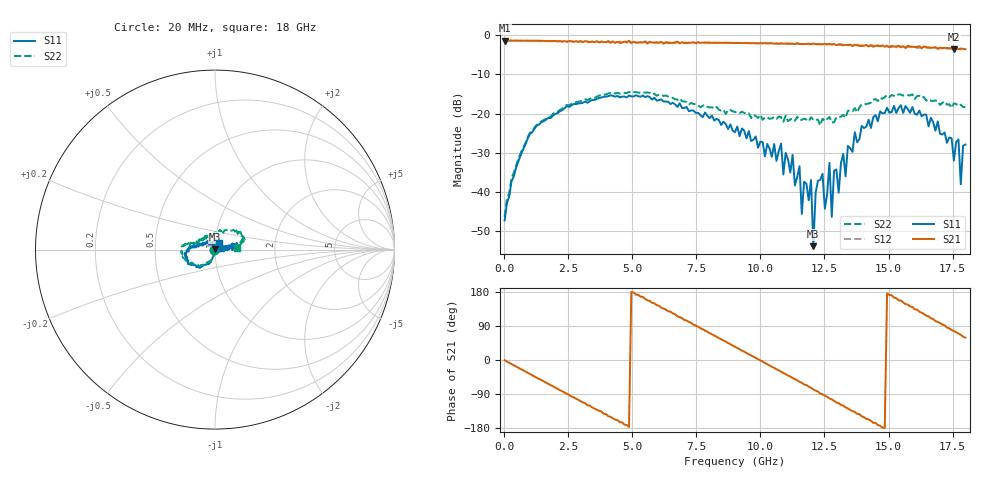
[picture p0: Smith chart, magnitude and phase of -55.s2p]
!Agilent Technologies,N5230A,US43500223,A.07.50.48
!Agilent N5230A: A.07.50.48
!Date: Sunday, January 31, 2016 13:36:31
!Correction: S11(Full 2 Port(1,2))
!S21(Full 2 Port(1,2))
!S12(Full 2 Port(1,2))
!S22(Full 2 Port(1,2))
!S2P File: Measurements: S11, S21, S12, S22:
# Hz S  RI  R 50
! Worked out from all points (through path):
!   201 points, 20 MHz to 18 GHz, reference 50 ohm
!   highest |S21| = -1.32 dB at 20 MHz (marker M1); lowest = -3.6 dB at 17.55 GHz (marker M2)
!   group delay of S21, straight-line fit = 102 ps
!   lowest |S11| = -53.9 dB at 12.07 GHz (marker M3), VSWR 1.00, Z = 49.8 + j0.117 ohm
!   |S11| at or under -10 dB: start of sweep to end of sweep
!   |S22| runs from -46.4 to -14.5 dB; largest |S21 - S12| = 0.077
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2e7  -0.00349 -0.0025  0.859 -0.0113  0.8605 -0.0142  -0.00469 -0.00101
1.0089e9  -0.0166 -0.0525  0.678 -0.5131  0.6764 -0.5149  -0.0171 -0.0541
3.0766e9  -0.0983 -0.0962  -0.3064 -0.759  -0.3201 -0.7628  -0.1247 -0.0772
6.0433e9  -0.1483 0.00658  -0.6466 0.4833  -0.6178 0.4968  -0.1726 0.0232
9.01e9  -0.0414 0.0401  0.6563 0.4582  0.6744 0.4338  -0.0957 0.0436
1.12575e10  0.0141 0.0261  0.5291 -0.5742  0.4974 -0.6035  -0.0459 0.0728
1.15272e10  -0.000936 0.0212  0.4165 -0.6539  0.3888 -0.6794  -0.0414 0.0714
1.16171e10  4.4e-05 0.0052  0.384 -0.6723  0.3423 -0.69  -0.0471 0.0684
1.19767e10  0.013 0.00541  0.2195 -0.739  0.1854 -0.7496  -0.0458 0.0773
1.20666e10  -0.00163 0.00118  0.167 -0.7685  0.1321 -0.7647  -0.0353 0.0753
1.22464e10  0.0124 0.00601  0.0891 -0.7691  0.0505 -0.7681  -0.0333 0.077
1.25161e10  -0.000176 0.00605  -0.0569 -0.7774  -0.0881 -0.7602  -0.0187 0.0779
1.26959e10  0.0201 -0.0121  -0.1503 -0.7608  -0.1919 -0.7475  -0.0232 0.0874
1.27858e10  0.00386 0.00279  -0.1849 -0.7414  -0.2245 -0.7286  -0.0151 0.075
1.28757e10  0.0066 -0.0173  -0.234 -0.7376  -0.2664 -0.7209  -0.0115 0.0769
1.30555e10  0.00962 0.00125  -0.3079 -0.7032  -0.3406 -0.6645  -0.00156 0.0914
1.36848e10  0.0577 -0.00302  -0.5584 -0.5165  -0.5701 -0.4842  0.0368 0.1113
1.50333e10  0.0972 0.0329  -0.6954 0.1052  -0.6979 0.1528  0.1312 0.095
1.75505e10  0.0244 0.00565  0.1559 0.6433  0.2109 0.6325  0.133 0.0215
1.77303e10  0.0427 0.0188  0.2367 0.6247  0.2894 0.6072  0.1232 0.0184
1.78202e10  0.012 0.00345  0.2712 0.6212  0.3172 0.5797  0.1278 0.0235
1.8e10  0.0208 0.0344  0.3425 0.5701  0.3865 0.5328  0.121 0.00876
